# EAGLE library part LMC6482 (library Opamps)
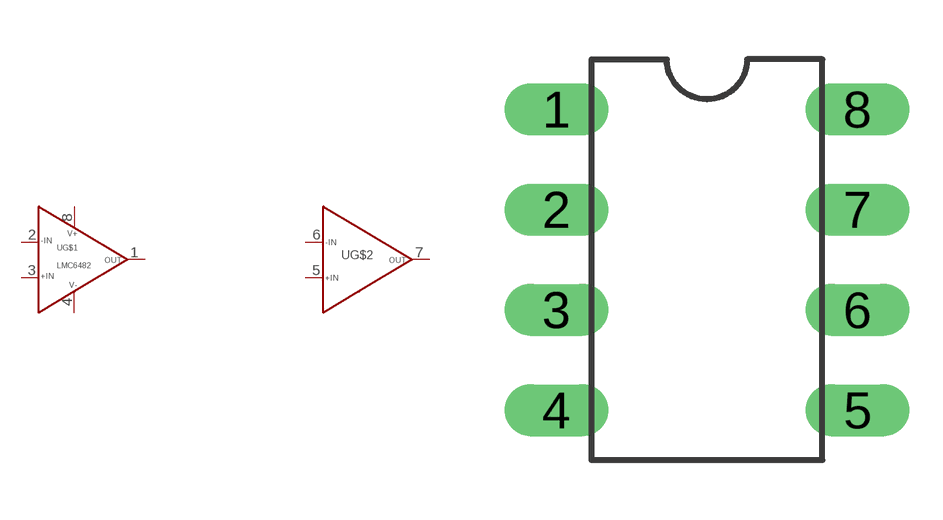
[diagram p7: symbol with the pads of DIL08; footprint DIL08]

Designator prefix -; gates G$1=CH1 G$2=CHGEN

## LMC6482  [DIL08]
1  G$1:OUTA
2  G$1:-INA
3  G$1:+INA
4  G$1:GND
5  G$2:+INB
6  G$2:-INB
7  G$2:OUTB
8  G$1:VCC

## Footprint DIL08 (pad centres in mm)
drill 0.813 long: 1 -3.81,3.81; 2 -3.81,1.27; 3 -3.81,-1.27; 4 -3.81,-3.81; 5 3.81,-3.81; 6 3.81,-1.27; 7 3.81,1.27; 8 3.81,3.81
